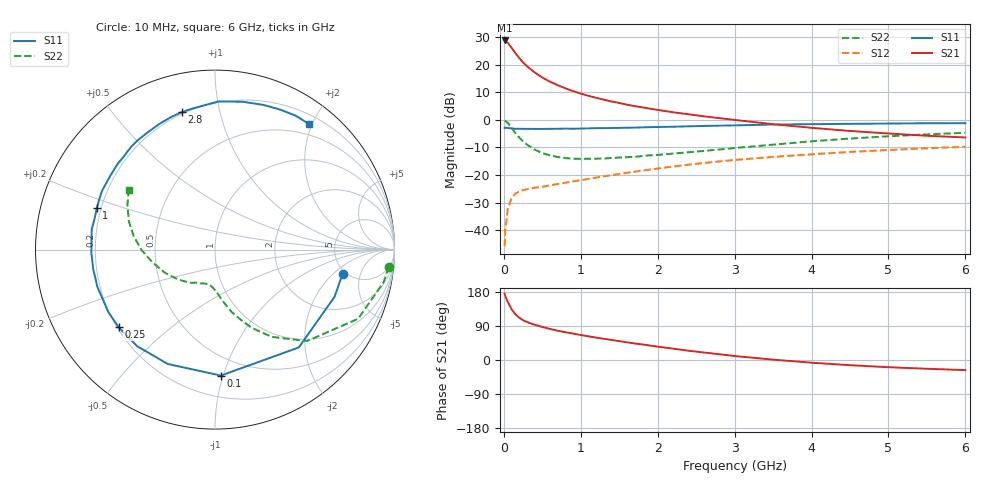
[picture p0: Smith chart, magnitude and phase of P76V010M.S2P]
! SIEMENS Small Signal Semiconductors
! BFP196
! Si NPN RF Bipolar Junction Transistor in SOT143
! VCE = 6 V  IC = 10 mA
! Common Emitter S-Parameters:  May  1996
# GHz  S  MA  R  50
!  f  S11  S21  S12  S22
! GHz  MAG  ANG  MAG  ANG  MAG  ANG  MAG  ANG
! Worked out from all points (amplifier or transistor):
!   36 points, 10 MHz to 6 GHz, reference 50 ohm
!   highest |S21| = 28.9 dB at 10 MHz (marker M1)
!   |S21| within 3 dB of that: start of sweep to 109.7 MHz
!   unconditionally stable (mu >= 1): 896 MHz to 3.263 GHz
!   at 250 MHz: K = 0.39, MSG = 23.2 dB, |S12| = -25.5 dB
!   at 1.4 GHz: K = 1.14, MAG = 11.1 dB, |S12| = -20.1 dB
!   at 6 GHz: K = 0.95, MSG = 1.7 dB, |S12| = -9.8 dB
!   S11 on the Smith chart (normalised r, x): 10 MHz: 4.69, -2.64; 100 MHz: 0.35, -0.98; 250 MHz: 0.21, -0.34; 1 GHz: 0.18, +0.17; 2.8 GHz: 0.19, +0.77; 6 GHz: 0.33, +1.96
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0.01  0.7235 -10.7  27.79 175.1  0.0051 88.2  0.9725 -5.7
0.02  0.7163 -21.5  27.24 168.5  0.0103 80.2  0.9569 -10.9
0.05  0.7178 -49.4  25.26 153.7  0.0235 67.4  0.8859 -25.8
0.1  0.7026 -87.3  20.57 134.2  0.0382 52.5  0.7228 -44.8
0.15  0.6896 -112.5  16.35 120.6  0.0459 42.5  0.5797 -57.0
0.2  0.6912 -129.0  13.36 111.8  0.0502 38.0  0.4802 -65.0
0.25  0.6892 -141.2  11.08 105.1  0.0532 34.9  0.4069 -70.6
0.3  0.6888 -149.7  9.489 100.2  0.0551 33.9  0.3581 -75.2
0.4  0.6874 -162.4  7.32 93.0  0.0586 33.3  0.2896 -81.5
0.5  0.6871 -170.9  5.888 87.2  0.0612 33.8  0.2502 -85.8
0.6  0.6892 -178.6  4.954 82.0  0.0649 35.0  0.2275 -89.6
0.7  0.6907 175.4  4.285 77.3  0.0687 36.7  0.2129 -93.0
0.8  0.6963 170.5  3.752 73.4  0.0725 37.9  0.2034 -96.6
1  0.6979 160.6  3.012 66.0  0.0806 40.6  0.1965 -101.6
1.1  0.7032 156.6  2.746 62.5  0.0849 41.3  0.1971 -104.3
1.6  0.7233 138.2  1.893 46.7  0.1097 43.6  0.211 -118.1
2.2  0.7532 119.9  1.38 30.0  0.1428 42.1  0.2452 -133.7
2.8  0.7885 103.5  1.08 15.3  0.1764 37.7  0.2907 -150.5
3.5  0.8263 88.5  0.837 1.0  0.2132 30.6  0.3561 -168.6
4.5  0.8501 71.5  0.631 -13.7  0.2626 20.0  0.4591 170.6
5.5  0.8712 58.9  0.516 -23.1  0.3061 8.7  0.547 153.1
6  0.874 53.0  0.481 -26.7  0.3253 2.5  0.5847 145.3
